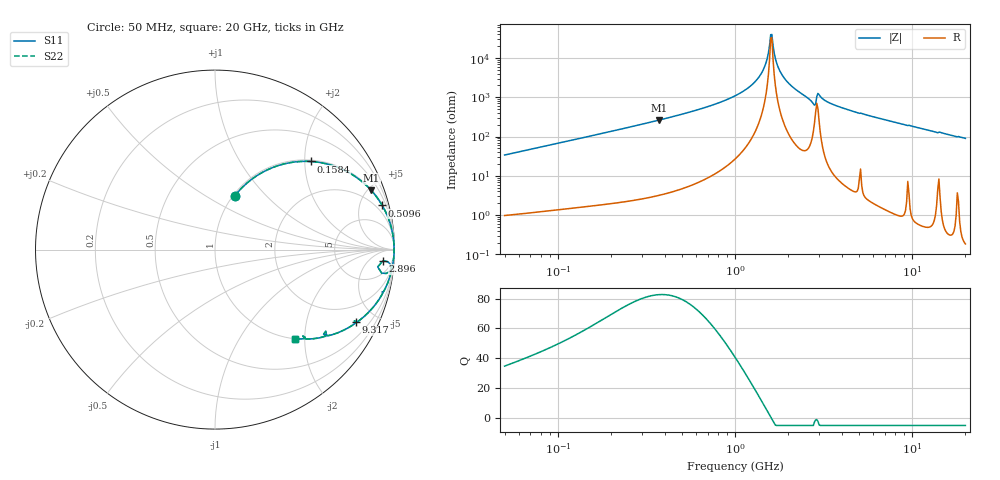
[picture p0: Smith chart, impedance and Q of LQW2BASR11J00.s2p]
!Murata Part Number: LQW2BASR11J00
!These Parameters are Measured in Series Mode Connection
!  o--[Z]--o
!Port1  Port2
!  o-------o
!Freq. Start=50[MHz] Stop=20[GHz], 401[Steps]
# Hz S RI R 50
!Freq.(Hz) S11(Real) S11(Imag) S21(Real) S21(Imag) S12(Real) S12(Imag) S22(Real) S22(Imag)
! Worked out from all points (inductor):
!   401 points, 50 MHz to 20 GHz, reference 50 ohm
!   read as one part in series: L = 107 nH near 51.52 MHz
!   highest Q = 82.6 at 372.1 MHz (marker M1), where L = 112 nH
!   self-resonance near 1.591 GHz
!   S11 on the Smith chart (normalised r, x): 50 MHz: 1.02, +0.68; 158.4 MHz: 1.03, +2.14; 509.6 MHz: 1.10, +7.55; 2.896 GHz: 15, -15; 9.317 GHz: 1.04, -3.87; 20 GHz: 1.00, -1.80
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5e7  0.1097 0.2985  0.8903 -0.2985  0.8903 -0.2985  0.1097 0.2985
1.364002e8  0.4596 0.4898  0.5404 -0.4898  0.5404 -0.4898  0.4596 0.4898
1.584406e8  0.5338 0.4909  0.4662 -0.4909  0.4662 -0.4909  0.5338 0.4909
3.721004e8  0.8701 0.3302  0.1299 -0.3302  0.1299 -0.3302  0.8701 0.3302
5.096456e8  0.9318 0.2459  0.0682 -0.2459  0.0682 -0.2459  0.9318 0.2459
1e9  0.9894 0.0909  0.0106 -0.0909  0.0106 -0.0909  0.9894 0.0909
1.196911e9  0.9948 0.0554  0.00524 -0.0554  0.00524 -0.0554  0.9948 0.0554
1.369645e9  0.997 0.0297  0.00299 -0.0297  0.00299 -0.0297  0.997 0.0297
1.476162e9  0.9977 0.0156  0.00233 -0.0156  0.00233 -0.0156  0.9977 0.0156
1.567309e9  0.9979 0.00427  0.00211 -0.00427  0.00211 -0.00427  0.9979 0.00427
1.614971e9  0.9979 -0.00139  0.00209 0.00139  0.00209 0.00139  0.9979 -0.00139
1.639343e9  0.9979 -0.00423  0.00211 0.00423  0.00211 0.00423  0.9979 -0.00423
1.740566e9  0.9977 -0.0156  0.00235 0.0156  0.00235 0.0156  0.9977 -0.0156
1.875929e9  0.9969 -0.0301  0.00305 0.0301  0.00305 0.0301  0.9969 -0.0301
2.114743e9  0.9947 -0.0541  0.00527 0.0541  0.00527 0.0541  0.9947 -0.0541
2.728004e9  0.9675 -0.1258  0.0325 0.1258  0.0325 0.1258  0.9675 -0.1258
2.896447e9  0.935 -0.0625  0.065 0.0625  0.065 0.0625  0.935 -0.0625
2.98453e9  0.9754 -0.0804  0.0246 0.0804  0.0246 0.0804  0.9754 -0.0804
3.850025e9  0.9689 -0.167  0.0311 0.167  0.0311 0.167  0.9689 -0.167
7.442007e9  0.8615 -0.3431  0.1385 0.3431  0.1385 0.3431  0.8615 -0.3431
9.316812e9  0.7863 -0.4042  0.2137 0.4042  0.2137 0.4042  0.7863 -0.4042
2e10  0.4473 -0.4962  0.5527 0.4962  0.5527 0.4962  0.4473 -0.4962
